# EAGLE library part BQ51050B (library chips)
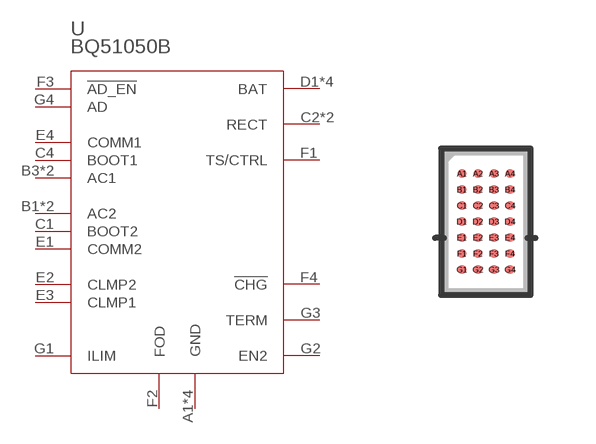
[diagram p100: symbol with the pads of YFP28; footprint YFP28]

Designator prefix U

## BQ51050B (BUILT_BY: EMA_UL_Team; MANUFACTURER_PART_NUMBER: BQ51050BYFPR; VENDOR: Texas Instruments)  [YFP28]
A1  GND  pwr
A2  GND  pwr
A3  GND  pwr
A4  GND  pwr
B1  AC2  in
B2  AC2  in
B3  AC1  in
B4  AC1  in
C1  BOOT2  out
C2  RECT  out
C3  RECT  out
C4  BOOT1  out
D1  BAT  out
D2  BAT  out
D3  BAT  out
D4  BAT  out
E1  COMM2  out
E2  CLMP2  out
E3  CLMP1  out
E4  COMM1  out
F1  TS/CTRL  in
F2  FOD  in
F3  !AD_EN  out
F4  !CHG  out
G1  ILIM
G2  EN2  in
G3  TERM  in
G4  AD  in

## Footprint YFP28 (pad centres in mm)
smd 0.229 x 0.229: A1 -0.6,1.2; A2 -0.2,1.2; A3 0.2,1.2; A4 0.6,1.2; B1 -0.6,0.8; B2 -0.2,0.8; B3 0.2,0.8; B4 0.6,0.8; C1 -0.6,0.4; C2 -0.2,0.4; C3 0.2,0.4; C4 0.6,0.4; D1 -0.6,0; D2 -0.2,0; D3 0.2,0; D4 0.6,0; E1 -0.6,-0.4; E2 -0.2,-0.4; E3 0.2,-0.4; E4 0.6,-0.4; F1 -0.6,-0.8; F2 -0.2,-0.8; F3 0.2,-0.8; F4 0.6,-0.8; G1 -0.6,-1.2; G2 -0.2,-1.2; G3 0.2,-1.2; G4 0.6,-1.2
